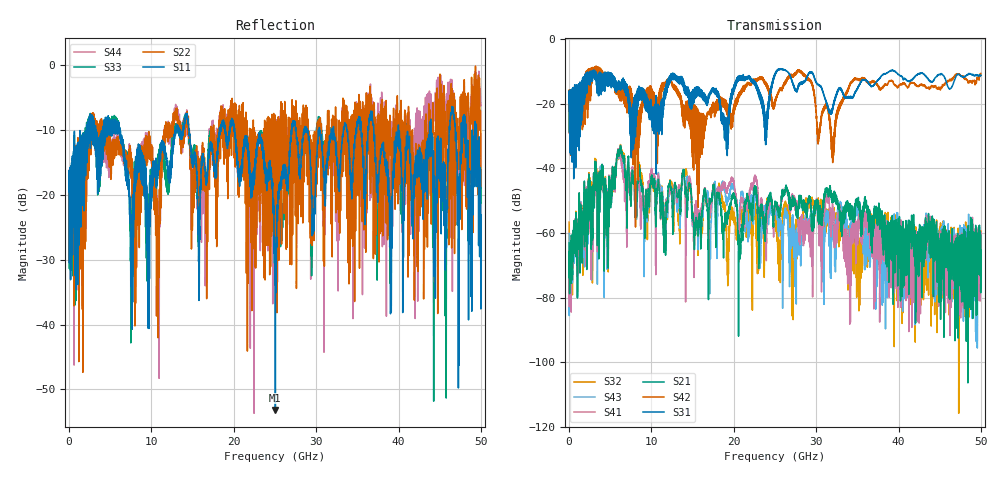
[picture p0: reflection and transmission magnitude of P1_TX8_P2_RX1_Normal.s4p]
!Keysight Technologies,N5225B,MY57041031,A.13.20.10
!Date: Friday, May 31, 2019 11:28:52
!Correction: S11(Full 4 Port(1,2,3,4))
!S12(Full 4 Port(1,2,3,4))
!S13(Full 4 Port(1,2,3,4))
!S14(Full 4 Port(1,2,3,4))
!S21(Full 4 Port(1,2,3,4))
!S22(Full 4 Port(1,2,3,4))
!S23(Full 4 Port(1,2,3,4))
!S24(Full 4 Port(1,2,3,4))
!S31(Full 4 Port(1,2,3,4))
!S32(Full 4 Port(1,2,3,4))
!S33(Full 4 Port(1,2,3,4))
!S34(Full 4 Port(1,2,3,4))
!S41(Full 4 Port(1,2,3,4))
!S42(Full 4 Port(1,2,3,4))
!S43(Full 4 Port(1,2,3,4))
!S44(Full 4 Port(1,2,3,4))
!S4P File: Measurements: <S11,S12,S13,S14>,
!<S21,S22,S23,S24>,
!<S31,S32,S33,S34>,
!<S41,S42,S43,S44>:
# Hz S  dB  R 50.0
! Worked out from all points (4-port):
!   5000 points, 10 MHz to 50 GHz, reference 50 ohm
!   strongest paths, dB at 10 MHz, 12.51 GHz, 25.01 GHz, 37.51 GHz, 50 GHz:
!     S31: -19.7, -10.8, -11.0, -12.6, -11.2
!     S42: -19.4, -14.2, -20.0, -14.7, -10.6
!     S21: -63.1, -50.2, -50.1, -54.8, -65.3
!     S41: -69.8, -50.1, -51.1, -60.0, -64.4
!     S43: -60.2, -47.9, -53.0, -69.3, -64.7
!     S32: -56.6, -46.0, -53.9, -58.9, -59.4
!   lowest |S11| = -53.2 dB at 25.05 GHz (marker M1), VSWR 1.00, Z = 49.8 - j0.135 ohm
!   |S11| at or under -10 dB: 6.192 GHz to 12.89 GHz (6.695 GHz wide, 70.2 % of centre); 20.1 GHz to 26.99 GHz (6.89 GHz wide, 29.3 % of centre); 40 GHz to 43.76 GHz (3.76 GHz wide, 8.98 % of centre)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
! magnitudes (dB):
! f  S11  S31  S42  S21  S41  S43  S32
! 10 MHz  -19.5  -19.7  -19.4  -63.1  -69.8  -60.2  -56.6
! 6.3 GHz  -12.0  -14.5  -19.0  -33.6  -35.9  -35.6  -33.5
! 11.65 GHz  -12.6  -18.2  -14.0  -60.9  -57.9  -57.6  -58.1
! 25.05 GHz  -53.2  -10.5  -19.2  -51.1  -51.7  -53.9  -55.8
! 27.29 GHz  -8.5  -14.5  -11.3  -49.2  -48.4  -57.7  -63.9
! 32.01 GHz  -10.3  -21.4  -38.2  -49.3  -51.8  -56.2  -54.8
! 50 GHz  -23.0  -11.2  -10.6  -65.3  -64.4  -64.7  -59.4
